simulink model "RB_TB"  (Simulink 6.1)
settings: Solver=ode3  SolverMode=SingleTasking  StartTime=0  StopTime=1000  FixedStep=0.05  RelTol=1e-3
libraries: simulink x2
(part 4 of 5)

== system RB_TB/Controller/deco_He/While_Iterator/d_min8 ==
  note: Model: RB_TB/Controller/deco_He/While_Iterator/d_minX
  Pt_new : Inport  Port=1  LatchInput=off
  In1 : Inport  Port=2  LatchInput=off
  In2 : Inport  Port=3  LatchInput=off
  BC : BusCreator  DialogController=Simulink.DDGSource_Bus
  BS1 : BusSelector  DialogController=Simulink.DDGSource_Bus  OutputSignals=He_b,M0,He_k,Pt
  BS2 : BusSelector  DialogController=Simulink.DDGSource_Bus  OutputSignals=rate_asc,asc_time,while,cnc_He,Palv_next,Palv
  Mux2 : Mux  Inputs=6
  Product2 : Product
  Sum1 : Sum  Inputs=-+|
  Switch : Switch  Threshold=2
  Switch1 : Switch  Threshold=2
  fnc : Fcn  Expr=u(6)-u(5)*u(2)*(u(3)-1/u(1))-(u(6)-u(4)+u(5)*u(2)/u(1))*exp(-u(1)*u(3))
  prod : Gain  Gain=10
  bus1 : Outport
  d_min : Outport  Port=2
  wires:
  BS1/3 -> Mux2/1, BC/3  "<He_k>"
  BS1/1 -> prod/1, BC/1  "<He_b>"
  BS1/2 -> Sum1/1, BC/2  "<M0>"
  Mux2/1 -> fnc/1
  fnc/1 -> BC/4  "Pt_stop"
  BS2/2 -> Mux2/3  "<asc_time>"
  BS2/4 -> Mux2/5  "<cnc_He>"
  In1/1 -> BS1/1
  Sum1/1 -> Product2/2
  prod/1 -> Product2/1
  Product2/1 -> d_min/1
  BC/1 -> bus1/1
  Switch/1 -> Sum1/2, Mux2/4  "Pt"
  BS1/4 -> Switch/3  "<Pt>"
  Pt_new/1 -> Switch/1
  Switch1/1 -> Mux2/6
  BS2/6 -> Switch1/3  "<Palv>"
  BS2/3 -> Switch/2, Switch1/2  "<while>"
  BS2/5 -> Switch1/1  "<Palv_next>"
  In2/1 -> BS2/1
  BS2/1 -> Mux2/2  "<rate_asc>"

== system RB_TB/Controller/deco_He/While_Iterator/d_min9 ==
  note: Model: RB_TB/Controller/deco_He/While_Iterator/d_minX
  Pt_new : Inport  Port=1  LatchInput=off
  In1 : Inport  Port=2  LatchInput=off
  In2 : Inport  Port=3  LatchInput=off
  BC : BusCreator  DialogController=Simulink.DDGSource_Bus
  BS1 : BusSelector  DialogController=Simulink.DDGSource_Bus  OutputSignals=He_b,M0,He_k,Pt
  BS2 : BusSelector  DialogController=Simulink.DDGSource_Bus  OutputSignals=rate_asc,asc_time,while,cnc_He,Palv_next,Palv
  Mux2 : Mux  Inputs=6
  Product2 : Product
  Sum1 : Sum  Inputs=-+|
  Switch : Switch  Threshold=2
  Switch1 : Switch  Threshold=2
  fnc : Fcn  Expr=u(6)-u(5)*u(2)*(u(3)-1/u(1))-(u(6)-u(4)+u(5)*u(2)/u(1))*exp(-u(1)*u(3))
  prod : Gain  Gain=10
  bus1 : Outport
  d_min : Outport  Port=2
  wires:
  BS2/1 -> Mux2/2  "<rate_asc>"
  In2/1 -> BS2/1
  BS2/5 -> Switch1/1  "<Palv_next>"
  BS2/3 -> Switch1/2, Switch/2  "<while>"
  BS2/6 -> Switch1/3  "<Palv>"
  Switch1/1 -> Mux2/6
  Pt_new/1 -> Switch/1
  BS1/4 -> Switch/3  "<Pt>"
  Switch/1 -> Mux2/4, Sum1/2  "Pt"
  BC/1 -> bus1/1
  Product2/1 -> d_min/1
  prod/1 -> Product2/1
  Sum1/1 -> Product2/2
  In1/1 -> BS1/1
  BS2/4 -> Mux2/5  "<cnc_He>"
  BS2/2 -> Mux2/3  "<asc_time>"
  fnc/1 -> BC/4  "Pt_stop"
  Mux2/1 -> fnc/1
  BS1/2 -> BC/2, Sum1/1  "<M0>"
  BS1/1 -> BC/1, prod/1  "<He_b>"
  BS1/3 -> BC/3, Mux2/1  "<He_k>"

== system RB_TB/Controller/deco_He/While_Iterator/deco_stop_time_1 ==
  note: Model: RB_TB/Controller/deco_He/While_Iterator/deco_stop_time_X
  In1 : Inport  Port=1  LatchInput=off
  In2 : Inport  Port=2  LatchInput=off
  >10e-300 : Saturate  UpperLimit=inf  LowerLimit=10e-320
  >10e-320 : Switch  Threshold=10e-320
  BS1 : BusSelector  DialogController=Simulink.DDGSource_Bus  OutputSignals=He_k,Pt_stop,He_b,M0
  BS2 : BusSelector  DialogController=Simulink.DDGSource_Bus  OutputSignals=Pstop_next,Palv_next,stop_time
  Constant : Constant
  Mem : Memory  InheritSampleTime=on
  Mux1 : Mux  Inputs=2
  Mux2 : Mux
  Mux3 : Mux  Inputs=2
  Mux4 : Mux  Inputs=3
  Mux5 : Mux  Inputs=3
  fcn(14)1 : Fcn  Expr=log(u(1))
  fcn(14)2 : Fcn  Expr=u(1)-u(2)
  fcn(14)4 : Fcn  Expr=(u(2)-u(3))/u(1)
  fcn(14)5 : Fcn  Expr=-u(2)/u(1)
  fcn1 : Fcn  Expr=u(2)+u(3)/u(1)
  fcn2 : Fcn  Expr=u(3)+(u(2)-u(3))*exp(-u(1)*u(4))
  Pt_new : Outport
  deco_stop_time : Outport  Port=2
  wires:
  >10e-300/1 -> Mux5/1
  Mux5/1 -> fcn(14)4/1
  fcn(14)2/1 -> >10e-300/1
  Mux3/1 -> fcn(14)2/1
  BS2/1 -> Mux4/3  "<Pstop_next>"
  Constant/1 -> >10e-320/3
  fcn(14)4/1 -> >10e-320/1, >10e-320/2
  fcn(14)1/1 -> Mux1/2
  >10e-320/1 -> fcn(14)1/1
  Mux4/1 -> fcn1/1
  fcn(14)5/1 -> deco_stop_time/1  "deco_stop_time"
  fcn1/1 -> Mux5/2  "M_next"
  BS2/2 -> Mux3/2, Mux5/3, Mux2/3  "<Palv_next>"
  BS1/1 -> Mux1/1, Mux2/1  "<He_k>"
  Mux1/1 -> fcn(14)5/1
  BS1/4 -> Mux4/2  "<M0>"
  BS1/3 -> Mux4/1  "<He_b>"
  In1/1 -> BS1/1
  BS1/2 -> Mux3/1, Mux2/2  "<Pt_stop>"
  Mux2/1 -> fcn2/1
  fcn2/1 -> Mem/1
  BS2/3 -> Mux2/4  "<stop_time>"
  Mem/1 -> Pt_new/1
  In2/1 -> BS2/1

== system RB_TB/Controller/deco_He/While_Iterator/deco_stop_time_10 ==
  note: Model: RB_TB/Controller/deco_He/While_Iterator/deco_stop_time_X
  In1 : Inport  Port=1  LatchInput=off
  In2 : Inport  Port=2  LatchInput=off
  >10e-300 : Saturate  UpperLimit=inf  LowerLimit=10e-320
  >10e-320 : Switch  Threshold=10e-320
  BS1 : BusSelector  DialogController=Simulink.DDGSource_Bus  OutputSignals=He_k,Pt_stop,He_b,M0
  BS2 : BusSelector  DialogController=Simulink.DDGSource_Bus  OutputSignals=Pstop_next,Palv_next,stop_time
  Constant : Constant
  Mem : Memory  InheritSampleTime=on
  Mux1 : Mux  Inputs=2
  Mux2 : Mux
  Mux3 : Mux  Inputs=2
  Mux4 : Mux  Inputs=3
  Mux5 : Mux  Inputs=3
  fcn(14)1 : Fcn  Expr=log(u(1))
  fcn(14)2 : Fcn  Expr=u(1)-u(2)
  fcn(14)4 : Fcn  Expr=(u(2)-u(3))/u(1)
  fcn(14)5 : Fcn  Expr=-u(2)/u(1)
  fcn1 : Fcn  Expr=u(2)+u(3)/u(1)
  fcn2 : Fcn  Expr=u(3)+(u(2)-u(3))*exp(-u(1)*u(4))
  Pt_new : Outport
  deco_stop_time : Outport  Port=2
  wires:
  >10e-300/1 -> Mux5/1
  Mux5/1 -> fcn(14)4/1
  fcn(14)2/1 -> >10e-300/1
  Mux3/1 -> fcn(14)2/1
  BS2/1 -> Mux4/3  "<Pstop_next>"
  Constant/1 -> >10e-320/3
  fcn(14)4/1 -> >10e-320/1, >10e-320/2
  fcn(14)1/1 -> Mux1/2
  >10e-320/1 -> fcn(14)1/1
  Mux4/1 -> fcn1/1
  fcn(14)5/1 -> deco_stop_time/1  "deco_stop_time"
  fcn1/1 -> Mux5/2  "M_next"
  BS2/2 -> Mux3/2, Mux5/3, Mux2/3  "<Palv_next>"
  BS1/1 -> Mux1/1, Mux2/1  "<He_k>"
  Mux1/1 -> fcn(14)5/1
  BS1/4 -> Mux4/2  "<M0>"
  BS1/3 -> Mux4/1  "<He_b>"
  In1/1 -> BS1/1
  BS1/2 -> Mux3/1, Mux2/2  "<Pt_stop>"
  Mux2/1 -> fcn2/1
  fcn2/1 -> Mem/1
  BS2/3 -> Mux2/4  "<stop_time>"
  Mem/1 -> Pt_new/1
  In2/1 -> BS2/1

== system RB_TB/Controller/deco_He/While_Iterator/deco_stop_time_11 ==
  note: Model: RB_TB/Controller/deco_He/While_Iterator/deco_stop_time_X
  In1 : Inport  Port=1  LatchInput=off
  In2 : Inport  Port=2  LatchInput=off
  >10e-300 : Saturate  UpperLimit=inf  LowerLimit=10e-320
  >10e-320 : Switch  Threshold=10e-320
  BS1 : BusSelector  DialogController=Simulink.DDGSource_Bus  OutputSignals=He_k,Pt_stop,He_b,M0
  BS2 : BusSelector  DialogController=Simulink.DDGSource_Bus  OutputSignals=Pstop_next,Palv_next,stop_time
  Constant : Constant
  Mem : Memory  InheritSampleTime=on
  Mux1 : Mux  Inputs=2
  Mux2 : Mux
  Mux3 : Mux  Inputs=2
  Mux4 : Mux  Inputs=3
  Mux5 : Mux  Inputs=3
  fcn(14)1 : Fcn  Expr=log(u(1))
  fcn(14)2 : Fcn  Expr=u(1)-u(2)
  fcn(14)4 : Fcn  Expr=(u(2)-u(3))/u(1)
  fcn(14)5 : Fcn  Expr=-u(2)/u(1)
  fcn1 : Fcn  Expr=u(2)+u(3)/u(1)
  fcn2 : Fcn  Expr=u(3)+(u(2)-u(3))*exp(-u(1)*u(4))
  Pt_new : Outport
  deco_stop_time : Outport  Port=2
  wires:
  In2/1 -> BS2/1
  Mem/1 -> Pt_new/1
  BS2/3 -> Mux2/4  "<stop_time>"
  fcn2/1 -> Mem/1
  Mux2/1 -> fcn2/1
  BS1/2 -> Mux2/2, Mux3/1  "<Pt_stop>"
  In1/1 -> BS1/1
  BS1/3 -> Mux4/1  "<He_b>"
  BS1/4 -> Mux4/2  "<M0>"
  Mux1/1 -> fcn(14)5/1
  BS1/1 -> Mux2/1, Mux1/1  "<He_k>"
  BS2/2 -> Mux2/3, Mux5/3, Mux3/2  "<Palv_next>"
  fcn1/1 -> Mux5/2  "M_next"
  fcn(14)5/1 -> deco_stop_time/1  "deco_stop_time"
  Mux4/1 -> fcn1/1
  >10e-320/1 -> fcn(14)1/1
  fcn(14)1/1 -> Mux1/2
  fcn(14)4/1 -> >10e-320/2, >10e-320/1
  Constant/1 -> >10e-320/3
  BS2/1 -> Mux4/3  "<Pstop_next>"
  Mux3/1 -> fcn(14)2/1
  fcn(14)2/1 -> >10e-300/1
  Mux5/1 -> fcn(14)4/1
  >10e-300/1 -> Mux5/1

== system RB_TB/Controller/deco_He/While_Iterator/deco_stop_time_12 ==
  note: Model: RB_TB/Controller/deco_He/While_Iterator/deco_stop_time_X
  In1 : Inport  Port=1  LatchInput=off
  In2 : Inport  Port=2  LatchInput=off
  >10e-300 : Saturate  UpperLimit=inf  LowerLimit=10e-320
  >10e-320 : Switch  Threshold=10e-320
  BS1 : BusSelector  DialogController=Simulink.DDGSource_Bus  OutputSignals=He_k,Pt_stop,He_b,M0
  BS2 : BusSelector  DialogController=Simulink.DDGSource_Bus  OutputSignals=Pstop_next,Palv_next,stop_time
  Constant : Constant
  Mem : Memory  InheritSampleTime=on
  Mux1 : Mux  Inputs=2
  Mux2 : Mux
  Mux3 : Mux  Inputs=2
  Mux4 : Mux  Inputs=3
  Mux5 : Mux  Inputs=3
  fcn(14)1 : Fcn  Expr=log(u(1))
  fcn(14)2 : Fcn  Expr=u(1)-u(2)
  fcn(14)4 : Fcn  Expr=(u(2)-u(3))/u(1)
  fcn(14)5 : Fcn  Expr=-u(2)/u(1)
  fcn1 : Fcn  Expr=u(2)+u(3)/u(1)
  fcn2 : Fcn  Expr=u(3)+(u(2)-u(3))*exp(-u(1)*u(4))
  Pt_new : Outport
  deco_stop_time : Outport  Port=2
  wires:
  >10e-300/1 -> Mux5/1
  Mux5/1 -> fcn(14)4/1
  fcn(14)2/1 -> >10e-300/1
  Mux3/1 -> fcn(14)2/1
  BS2/1 -> Mux4/3  "<Pstop_next>"
  Constant/1 -> >10e-320/3
  fcn(14)4/1 -> >10e-320/1, >10e-320/2
  fcn(14)1/1 -> Mux1/2
  >10e-320/1 -> fcn(14)1/1
  Mux4/1 -> fcn1/1
  fcn(14)5/1 -> deco_stop_time/1  "deco_stop_time"
  fcn1/1 -> Mux5/2  "M_next"
  BS2/2 -> Mux3/2, Mux5/3, Mux2/3  "<Palv_next>"
  BS1/1 -> Mux1/1, Mux2/1  "<He_k>"
  Mux1/1 -> fcn(14)5/1
  BS1/4 -> Mux4/2  "<M0>"
  BS1/3 -> Mux4/1  "<He_b>"
  In1/1 -> BS1/1
  BS1/2 -> Mux3/1, Mux2/2  "<Pt_stop>"
  Mux2/1 -> fcn2/1
  fcn2/1 -> Mem/1
  BS2/3 -> Mux2/4  "<stop_time>"
  Mem/1 -> Pt_new/1
  In2/1 -> BS2/1

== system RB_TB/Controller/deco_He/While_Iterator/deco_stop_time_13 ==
  note: Model: RB_TB/Controller/deco_He/While_Iterator/deco_stop_time_X
  In1 : Inport  Port=1  LatchInput=off
  In2 : Inport  Port=2  LatchInput=off
  >10e-300 : Saturate  UpperLimit=inf  LowerLimit=10e-320
  >10e-320 : Switch  Threshold=10e-320
  BS1 : BusSelector  DialogController=Simulink.DDGSource_Bus  OutputSignals=He_k,Pt_stop,He_b,M0
  BS2 : BusSelector  DialogController=Simulink.DDGSource_Bus  OutputSignals=Pstop_next,Palv_next,stop_time
  Constant : Constant
  Mem : Memory  InheritSampleTime=on
  Mux1 : Mux  Inputs=2
  Mux2 : Mux
  Mux3 : Mux  Inputs=2
  Mux4 : Mux  Inputs=3
  Mux5 : Mux  Inputs=3
  fcn(14)1 : Fcn  Expr=log(u(1))
  fcn(14)2 : Fcn  Expr=u(1)-u(2)
  fcn(14)4 : Fcn  Expr=(u(2)-u(3))/u(1)
  fcn(14)5 : Fcn  Expr=-u(2)/u(1)
  fcn1 : Fcn  Expr=u(2)+u(3)/u(1)
  fcn2 : Fcn  Expr=u(3)+(u(2)-u(3))*exp(-u(1)*u(4))
  Pt_new : Outport
  deco_stop_time : Outport  Port=2
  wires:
  In2/1 -> BS2/1
  Mem/1 -> Pt_new/1
  BS2/3 -> Mux2/4  "<stop_time>"
  fcn2/1 -> Mem/1
  Mux2/1 -> fcn2/1
  BS1/2 -> Mux2/2, Mux3/1  "<Pt_stop>"
  In1/1 -> BS1/1
  BS1/3 -> Mux4/1  "<He_b>"
  BS1/4 -> Mux4/2  "<M0>"
  Mux1/1 -> fcn(14)5/1
  BS1/1 -> Mux2/1, Mux1/1  "<He_k>"
  BS2/2 -> Mux2/3, Mux5/3, Mux3/2  "<Palv_next>"
  fcn1/1 -> Mux5/2  "M_next"
  fcn(14)5/1 -> deco_stop_time/1  "deco_stop_time"
  Mux4/1 -> fcn1/1
  >10e-320/1 -> fcn(14)1/1
  fcn(14)1/1 -> Mux1/2
  fcn(14)4/1 -> >10e-320/2, >10e-320/1
  Constant/1 -> >10e-320/3
  BS2/1 -> Mux4/3  "<Pstop_next>"
  Mux3/1 -> fcn(14)2/1
  fcn(14)2/1 -> >10e-300/1
  Mux5/1 -> fcn(14)4/1
  >10e-300/1 -> Mux5/1

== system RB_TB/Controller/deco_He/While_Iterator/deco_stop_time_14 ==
  note: Model: RB_TB/Controller/deco_He/While_Iterator/deco_stop_time_X
  In1 : Inport  Port=1  LatchInput=off
  In2 : Inport  Port=2  LatchInput=off
  >10e-300 : Saturate  UpperLimit=inf  LowerLimit=10e-320
  >10e-320 : Switch  Threshold=10e-320
  BS1 : BusSelector  DialogController=Simulink.DDGSource_Bus  OutputSignals=He_k,Pt_stop,He_b,M0
  BS2 : BusSelector  DialogController=Simulink.DDGSource_Bus  OutputSignals=Pstop_next,Palv_next,stop_time
  Constant : Constant
  Mem : Memory  InheritSampleTime=on
  Mux1 : Mux  Inputs=2
  Mux2 : Mux
  Mux3 : Mux  Inputs=2
  Mux4 : Mux  Inputs=3
  Mux5 : Mux  Inputs=3
  fcn(14)1 : Fcn  Expr=log(u(1))
  fcn(14)2 : Fcn  Expr=u(1)-u(2)
  fcn(14)4 : Fcn  Expr=(u(2)-u(3))/u(1)
  fcn(14)5 : Fcn  Expr=-u(2)/u(1)
  fcn1 : Fcn  Expr=u(2)+u(3)/u(1)
  fcn2 : Fcn  Expr=u(3)+(u(2)-u(3))*exp(-u(1)*u(4))
  Pt_new : Outport
  deco_stop_time : Outport  Port=2
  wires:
  >10e-300/1 -> Mux5/1
  Mux5/1 -> fcn(14)4/1
  fcn(14)2/1 -> >10e-300/1
  Mux3/1 -> fcn(14)2/1
  BS2/1 -> Mux4/3  "<Pstop_next>"
  Constant/1 -> >10e-320/3
  fcn(14)4/1 -> >10e-320/1, >10e-320/2
  fcn(14)1/1 -> Mux1/2
  >10e-320/1 -> fcn(14)1/1
  Mux4/1 -> fcn1/1
  fcn(14)5/1 -> deco_stop_time/1  "deco_stop_time"
  fcn1/1 -> Mux5/2  "M_next"
  BS2/2 -> Mux3/2, Mux5/3, Mux2/3  "<Palv_next>"
  BS1/1 -> Mux1/1, Mux2/1  "<He_k>"
  Mux1/1 -> fcn(14)5/1
  BS1/4 -> Mux4/2  "<M0>"
  BS1/3 -> Mux4/1  "<He_b>"
  In1/1 -> BS1/1
  BS1/2 -> Mux3/1, Mux2/2  "<Pt_stop>"
  Mux2/1 -> fcn2/1
  fcn2/1 -> Mem/1
  BS2/3 -> Mux2/4  "<stop_time>"
  Mem/1 -> Pt_new/1
  In2/1 -> BS2/1

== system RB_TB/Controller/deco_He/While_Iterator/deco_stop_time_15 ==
  note: Model: RB_TB/Controller/deco_He/While_Iterator/deco_stop_time_X
  In1 : Inport  Port=1  LatchInput=off
  In2 : Inport  Port=2  LatchInput=off
  >10e-300 : Saturate  UpperLimit=inf  LowerLimit=10e-320
  >10e-320 : Switch  Threshold=10e-320
  BS1 : BusSelector  DialogController=Simulink.DDGSource_Bus  OutputSignals=He_k,Pt_stop,He_b,M0
  BS2 : BusSelector  DialogController=Simulink.DDGSource_Bus  OutputSignals=Pstop_next,Palv_next,stop_time
  Constant : Constant
  Mem : Memory  InheritSampleTime=on
  Mux1 : Mux  Inputs=2
  Mux2 : Mux
  Mux3 : Mux  Inputs=2
  Mux4 : Mux  Inputs=3
  Mux5 : Mux  Inputs=3
  fcn(14)1 : Fcn  Expr=log(u(1))
  fcn(14)2 : Fcn  Expr=u(1)-u(2)
  fcn(14)4 : Fcn  Expr=(u(2)-u(3))/u(1)
  fcn(14)5 : Fcn  Expr=-u(2)/u(1)
  fcn1 : Fcn  Expr=u(2)+u(3)/u(1)
  fcn2 : Fcn  Expr=u(3)+(u(2)-u(3))*exp(-u(1)*u(4))
  Pt_new : Outport
  deco_stop_time : Outport  Port=2
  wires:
  In2/1 -> BS2/1
  Mem/1 -> Pt_new/1
  BS2/3 -> Mux2/4  "<stop_time>"
  fcn2/1 -> Mem/1
  Mux2/1 -> fcn2/1
  BS1/2 -> Mux2/2, Mux3/1  "<Pt_stop>"
  In1/1 -> BS1/1
  BS1/3 -> Mux4/1  "<He_b>"
  BS1/4 -> Mux4/2  "<M0>"
  Mux1/1 -> fcn(14)5/1
  BS1/1 -> Mux2/1, Mux1/1  "<He_k>"
  BS2/2 -> Mux2/3, Mux5/3, Mux3/2  "<Palv_next>"
  fcn1/1 -> Mux5/2  "M_next"
  fcn(14)5/1 -> deco_stop_time/1  "deco_stop_time"
  Mux4/1 -> fcn1/1
  >10e-320/1 -> fcn(14)1/1
  fcn(14)1/1 -> Mux1/2
  fcn(14)4/1 -> >10e-320/2, >10e-320/1
  Constant/1 -> >10e-320/3
  BS2/1 -> Mux4/3  "<Pstop_next>"
  Mux3/1 -> fcn(14)2/1
  fcn(14)2/1 -> >10e-300/1
  Mux5/1 -> fcn(14)4/1
  >10e-300/1 -> Mux5/1

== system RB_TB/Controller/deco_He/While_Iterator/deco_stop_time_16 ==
  note: Model: RB_TB/Controller/deco_He/While_Iterator/deco_stop_time_X
  In1 : Inport  Port=1  LatchInput=off
  In2 : Inport  Port=2  LatchInput=off
  >10e-300 : Saturate  UpperLimit=inf  LowerLimit=10e-320
  >10e-320 : Switch  Threshold=10e-320
  BS1 : BusSelector  DialogController=Simulink.DDGSource_Bus  OutputSignals=He_k,Pt_stop,He_b,M0
  BS2 : BusSelector  DialogController=Simulink.DDGSource_Bus  OutputSignals=Pstop_next,Palv_next,stop_time
  Constant : Constant
  Mem : Memory  InheritSampleTime=on
  Mux1 : Mux  Inputs=2
  Mux2 : Mux
  Mux3 : Mux  Inputs=2
  Mux4 : Mux  Inputs=3
  Mux5 : Mux  Inputs=3
  fcn(14)1 : Fcn  Expr=log(u(1))
  fcn(14)2 : Fcn  Expr=u(1)-u(2)
  fcn(14)4 : Fcn  Expr=(u(2)-u(3))/u(1)
  fcn(14)5 : Fcn  Expr=-u(2)/u(1)
  fcn1 : Fcn  Expr=u(2)+u(3)/u(1)
  fcn2 : Fcn  Expr=u(3)+(u(2)-u(3))*exp(-u(1)*u(4))
  Pt_new : Outport
  deco_stop_time : Outport  Port=2
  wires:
  >10e-300/1 -> Mux5/1
  Mux5/1 -> fcn(14)4/1
  fcn(14)2/1 -> >10e-300/1
  Mux3/1 -> fcn(14)2/1
  BS2/1 -> Mux4/3  "<Pstop_next>"
  Constant/1 -> >10e-320/3
  fcn(14)4/1 -> >10e-320/1, >10e-320/2
  fcn(14)1/1 -> Mux1/2
  >10e-320/1 -> fcn(14)1/1
  Mux4/1 -> fcn1/1
  fcn(14)5/1 -> deco_stop_time/1  "deco_stop_time"
  fcn1/1 -> Mux5/2  "M_next"
  BS2/2 -> Mux3/2, Mux5/3, Mux2/3  "<Palv_next>"
  BS1/1 -> Mux1/1, Mux2/1  "<He_k>"
  Mux1/1 -> fcn(14)5/1
  BS1/4 -> Mux4/2  "<M0>"
  BS1/3 -> Mux4/1  "<He_b>"
  In1/1 -> BS1/1
  BS1/2 -> Mux3/1, Mux2/2  "<Pt_stop>"
  Mux2/1 -> fcn2/1
  fcn2/1 -> Mem/1
  BS2/3 -> Mux2/4  "<stop_time>"
  Mem/1 -> Pt_new/1
  In2/1 -> BS2/1

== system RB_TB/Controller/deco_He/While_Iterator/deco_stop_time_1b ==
  note: Model: RB_TB/Controller/deco_He/While_Iterator/deco_stop_time_X
  In1 : Inport  Port=1  LatchInput=off
  In2 : Inport  Port=2  LatchInput=off
  >10e-300 : Saturate  UpperLimit=inf  LowerLimit=10e-320
  >10e-320 : Switch  Threshold=10e-320
  BS1 : BusSelector  DialogController=Simulink.DDGSource_Bus  OutputSignals=He_k,Pt_stop,He_b,M0
  BS2 : BusSelector  DialogController=Simulink.DDGSource_Bus  OutputSignals=Pstop_next,Palv_next,stop_time
  Constant : Constant
  Mem : Memory  InheritSampleTime=on
  Mux1 : Mux  Inputs=2
  Mux2 : Mux
  Mux3 : Mux  Inputs=2
  Mux4 : Mux  Inputs=3
  Mux5 : Mux  Inputs=3
  fcn(14)1 : Fcn  Expr=log(u(1))
  fcn(14)2 : Fcn  Expr=u(1)-u(2)
  fcn(14)4 : Fcn  Expr=(u(2)-u(3))/u(1)
  fcn(14)5 : Fcn  Expr=-u(2)/u(1)
  fcn1 : Fcn  Expr=u(2)+u(3)/u(1)
  fcn2 : Fcn  Expr=u(3)+(u(2)-u(3))*exp(-u(1)*u(4))
  Pt_new : Outport
  deco_stop_time : Outport  Port=2
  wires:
  >10e-300/1 -> Mux5/1
  Mux5/1 -> fcn(14)4/1
  fcn(14)2/1 -> >10e-300/1
  Mux3/1 -> fcn(14)2/1
  BS2/1 -> Mux4/3  "<Pstop_next>"
  Constant/1 -> >10e-320/3
  fcn(14)4/1 -> >10e-320/1, >10e-320/2
  fcn(14)1/1 -> Mux1/2
  >10e-320/1 -> fcn(14)1/1
  Mux4/1 -> fcn1/1
  fcn(14)5/1 -> deco_stop_time/1  "deco_stop_time"
  fcn1/1 -> Mux5/2  "M_next"
  BS2/2 -> Mux3/2, Mux5/3, Mux2/3  "<Palv_next>"
  BS1/1 -> Mux1/1, Mux2/1  "<He_k>"
  Mux1/1 -> fcn(14)5/1
  BS1/4 -> Mux4/2  "<M0>"
  BS1/3 -> Mux4/1  "<He_b>"
  In1/1 -> BS1/1
  BS1/2 -> Mux3/1, Mux2/2  "<Pt_stop>"
  Mux2/1 -> fcn2/1
  fcn2/1 -> Mem/1
  BS2/3 -> Mux2/4  "<stop_time>"
  Mem/1 -> Pt_new/1
  In2/1 -> BS2/1

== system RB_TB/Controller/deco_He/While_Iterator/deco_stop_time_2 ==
  note: Model: RB_TB/Controller/deco_He/While_Iterator/deco_stop_time_X
  In1 : Inport  Port=1  LatchInput=off
  In2 : Inport  Port=2  LatchInput=off
  >10e-300 : Saturate  UpperLimit=inf  LowerLimit=10e-320
  >10e-320 : Switch  Threshold=10e-320
  BS1 : BusSelector  DialogController=Simulink.DDGSource_Bus  OutputSignals=He_k,Pt_stop,He_b,M0
  BS2 : BusSelector  DialogController=Simulink.DDGSource_Bus  OutputSignals=Pstop_next,Palv_next,stop_time
  Constant : Constant
  Mem : Memory  InheritSampleTime=on
  Mux1 : Mux  Inputs=2
  Mux2 : Mux
  Mux3 : Mux  Inputs=2
  Mux4 : Mux  Inputs=3
  Mux5 : Mux  Inputs=3
  fcn(14)1 : Fcn  Expr=log(u(1))
  fcn(14)2 : Fcn  Expr=u(1)-u(2)
  fcn(14)4 : Fcn  Expr=(u(2)-u(3))/u(1)
  fcn(14)5 : Fcn  Expr=-u(2)/u(1)
  fcn1 : Fcn  Expr=u(2)+u(3)/u(1)
  fcn2 : Fcn  Expr=u(3)+(u(2)-u(3))*exp(-u(1)*u(4))
  Pt_new : Outport
  deco_stop_time : Outport  Port=2
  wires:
  In2/1 -> BS2/1
  Mem/1 -> Pt_new/1
  BS2/3 -> Mux2/4  "<stop_time>"
  fcn2/1 -> Mem/1
  Mux2/1 -> fcn2/1
  BS1/2 -> Mux2/2, Mux3/1  "<Pt_stop>"
  In1/1 -> BS1/1
  BS1/3 -> Mux4/1  "<He_b>"
  BS1/4 -> Mux4/2  "<M0>"
  Mux1/1 -> fcn(14)5/1
  BS1/1 -> Mux2/1, Mux1/1  "<He_k>"
  BS2/2 -> Mux2/3, Mux5/3, Mux3/2  "<Palv_next>"
  fcn1/1 -> Mux5/2  "M_next"
  fcn(14)5/1 -> deco_stop_time/1  "deco_stop_time"
  Mux4/1 -> fcn1/1
  >10e-320/1 -> fcn(14)1/1
  fcn(14)1/1 -> Mux1/2
  fcn(14)4/1 -> >10e-320/2, >10e-320/1
  Constant/1 -> >10e-320/3
  BS2/1 -> Mux4/3  "<Pstop_next>"
  Mux3/1 -> fcn(14)2/1
  fcn(14)2/1 -> >10e-300/1
  Mux5/1 -> fcn(14)4/1
  >10e-300/1 -> Mux5/1

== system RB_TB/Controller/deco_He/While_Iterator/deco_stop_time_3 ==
  note: Model: RB_TB/Controller/deco_He/While_Iterator/deco_stop_time_X
  In1 : Inport  Port=1  LatchInput=off
  In2 : Inport  Port=2  LatchInput=off
  >10e-300 : Saturate  UpperLimit=inf  LowerLimit=10e-320
  >10e-320 : Switch  Threshold=10e-320
  BS1 : BusSelector  DialogController=Simulink.DDGSource_Bus  OutputSignals=He_k,Pt_stop,He_b,M0
  BS2 : BusSelector  DialogController=Simulink.DDGSource_Bus  OutputSignals=Pstop_next,Palv_next,stop_time
  Constant : Constant
  Mem : Memory  InheritSampleTime=on
  Mux1 : Mux  Inputs=2
  Mux2 : Mux
  Mux3 : Mux  Inputs=2
  Mux4 : Mux  Inputs=3
  Mux5 : Mux  Inputs=3
  fcn(14)1 : Fcn  Expr=log(u(1))
  fcn(14)2 : Fcn  Expr=u(1)-u(2)
  fcn(14)4 : Fcn  Expr=(u(2)-u(3))/u(1)
  fcn(14)5 : Fcn  Expr=-u(2)/u(1)
  fcn1 : Fcn  Expr=u(2)+u(3)/u(1)
  fcn2 : Fcn  Expr=u(3)+(u(2)-u(3))*exp(-u(1)*u(4))
  Pt_new : Outport
  deco_stop_time : Outport  Port=2
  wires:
  In2/1 -> BS2/1
  Mem/1 -> Pt_new/1
  BS2/3 -> Mux2/4  "<stop_time>"
  fcn2/1 -> Mem/1
  Mux2/1 -> fcn2/1
  BS1/2 -> Mux2/2, Mux3/1  "<Pt_stop>"
  In1/1 -> BS1/1
  BS1/3 -> Mux4/1  "<He_b>"
  BS1/4 -> Mux4/2  "<M0>"
  Mux1/1 -> fcn(14)5/1
  BS1/1 -> Mux2/1, Mux1/1  "<He_k>"
  BS2/2 -> Mux2/3, Mux5/3, Mux3/2  "<Palv_next>"
  fcn1/1 -> Mux5/2  "M_next"
  fcn(14)5/1 -> deco_stop_time/1  "deco_stop_time"
  Mux4/1 -> fcn1/1
  >10e-320/1 -> fcn(14)1/1
  fcn(14)1/1 -> Mux1/2
  fcn(14)4/1 -> >10e-320/2, >10e-320/1
  Constant/1 -> >10e-320/3
  BS2/1 -> Mux4/3  "<Pstop_next>"
  Mux3/1 -> fcn(14)2/1
  fcn(14)2/1 -> >10e-300/1
  Mux5/1 -> fcn(14)4/1
  >10e-300/1 -> Mux5/1

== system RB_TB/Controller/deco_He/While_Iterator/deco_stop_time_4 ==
  note: Model: RB_TB/Controller/deco_He/While_Iterator/deco_stop_time_X
  In1 : Inport  Port=1  LatchInput=off
  In2 : Inport  Port=2  LatchInput=off
  >10e-300 : Saturate  UpperLimit=inf  LowerLimit=10e-320
  >10e-320 : Switch  Threshold=10e-320
  BS1 : BusSelector  DialogController=Simulink.DDGSource_Bus  OutputSignals=He_k,Pt_stop,He_b,M0
  BS2 : BusSelector  DialogController=Simulink.DDGSource_Bus  OutputSignals=Pstop_next,Palv_next,stop_time
  Constant : Constant
  Mem : Memory  InheritSampleTime=on
  Mux1 : Mux  Inputs=2
  Mux2 : Mux
  Mux3 : Mux  Inputs=2
  Mux4 : Mux  Inputs=3
  Mux5 : Mux  Inputs=3
  fcn(14)1 : Fcn  Expr=log(u(1))
  fcn(14)2 : Fcn  Expr=u(1)-u(2)
  fcn(14)4 : Fcn  Expr=(u(2)-u(3))/u(1)
  fcn(14)5 : Fcn  Expr=-u(2)/u(1)
  fcn1 : Fcn  Expr=u(2)+u(3)/u(1)
  fcn2 : Fcn  Expr=u(3)+(u(2)-u(3))*exp(-u(1)*u(4))
  Pt_new : Outport
  deco_stop_time : Outport  Port=2
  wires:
  >10e-300/1 -> Mux5/1
  Mux5/1 -> fcn(14)4/1
  fcn(14)2/1 -> >10e-300/1
  Mux3/1 -> fcn(14)2/1
  BS2/1 -> Mux4/3  "<Pstop_next>"
  Constant/1 -> >10e-320/3
  fcn(14)4/1 -> >10e-320/1, >10e-320/2
  fcn(14)1/1 -> Mux1/2
  >10e-320/1 -> fcn(14)1/1
  Mux4/1 -> fcn1/1
  fcn(14)5/1 -> deco_stop_time/1  "deco_stop_time"
  fcn1/1 -> Mux5/2  "M_next"
  BS2/2 -> Mux3/2, Mux5/3, Mux2/3  "<Palv_next>"
  BS1/1 -> Mux1/1, Mux2/1  "<He_k>"
  Mux1/1 -> fcn(14)5/1
  BS1/4 -> Mux4/2  "<M0>"
  BS1/3 -> Mux4/1  "<He_b>"
  In1/1 -> BS1/1
  BS1/2 -> Mux3/1, Mux2/2  "<Pt_stop>"
  Mux2/1 -> fcn2/1
  fcn2/1 -> Mem/1
  BS2/3 -> Mux2/4  "<stop_time>"
  Mem/1 -> Pt_new/1
  In2/1 -> BS2/1

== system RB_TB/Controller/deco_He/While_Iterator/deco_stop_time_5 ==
  note: Model: RB_TB/Controller/deco_He/While_Iterator/deco_stop_time_X
  In1 : Inport  Port=1  LatchInput=off
  In2 : Inport  Port=2  LatchInput=off
  >10e-300 : Saturate  UpperLimit=inf  LowerLimit=10e-320
  >10e-320 : Switch  Threshold=10e-320
  BS1 : BusSelector  DialogController=Simulink.DDGSource_Bus  OutputSignals=He_k,Pt_stop,He_b,M0
  BS2 : BusSelector  DialogController=Simulink.DDGSource_Bus  OutputSignals=Pstop_next,Palv_next,stop_time
  Constant : Constant
  Mem : Memory  InheritSampleTime=on
  Mux1 : Mux  Inputs=2
  Mux2 : Mux
  Mux3 : Mux  Inputs=2
  Mux4 : Mux  Inputs=3
  Mux5 : Mux  Inputs=3
  fcn(14)1 : Fcn  Expr=log(u(1))
  fcn(14)2 : Fcn  Expr=u(1)-u(2)
  fcn(14)4 : Fcn  Expr=(u(2)-u(3))/u(1)
  fcn(14)5 : Fcn  Expr=-u(2)/u(1)
  fcn1 : Fcn  Expr=u(2)+u(3)/u(1)
  fcn2 : Fcn  Expr=u(3)+(u(2)-u(3))*exp(-u(1)*u(4))
  Pt_new : Outport
  deco_stop_time : Outport  Port=2
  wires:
  In2/1 -> BS2/1
  Mem/1 -> Pt_new/1
  BS2/3 -> Mux2/4  "<stop_time>"
  fcn2/1 -> Mem/1
  Mux2/1 -> fcn2/1
  BS1/2 -> Mux2/2, Mux3/1  "<Pt_stop>"
  In1/1 -> BS1/1
  BS1/3 -> Mux4/1  "<He_b>"
  BS1/4 -> Mux4/2  "<M0>"
  Mux1/1 -> fcn(14)5/1
  BS1/1 -> Mux2/1, Mux1/1  "<He_k>"
  BS2/2 -> Mux2/3, Mux5/3, Mux3/2  "<Palv_next>"
  fcn1/1 -> Mux5/2  "M_next"
  fcn(14)5/1 -> deco_stop_time/1  "deco_stop_time"
  Mux4/1 -> fcn1/1
  >10e-320/1 -> fcn(14)1/1
  fcn(14)1/1 -> Mux1/2
  fcn(14)4/1 -> >10e-320/2, >10e-320/1
  Constant/1 -> >10e-320/3
  BS2/1 -> Mux4/3  "<Pstop_next>"
  Mux3/1 -> fcn(14)2/1
  fcn(14)2/1 -> >10e-300/1
  Mux5/1 -> fcn(14)4/1
  >10e-300/1 -> Mux5/1

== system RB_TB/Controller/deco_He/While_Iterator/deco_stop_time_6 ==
  note: Model: RB_TB/Controller/deco_He/While_Iterator/deco_stop_time_X
  In1 : Inport  Port=1  LatchInput=off
  In2 : Inport  Port=2  LatchInput=off
  >10e-300 : Saturate  UpperLimit=inf  LowerLimit=10e-320
  >10e-320 : Switch  Threshold=10e-320
  BS1 : BusSelector  DialogController=Simulink.DDGSource_Bus  OutputSignals=He_k,Pt_stop,He_b,M0
  BS2 : BusSelector  DialogController=Simulink.DDGSource_Bus  OutputSignals=Pstop_next,Palv_next,stop_time
  Constant : Constant
  Mem : Memory  InheritSampleTime=on
  Mux1 : Mux  Inputs=2
  Mux2 : Mux
  Mux3 : Mux  Inputs=2
  Mux4 : Mux  Inputs=3
  Mux5 : Mux  Inputs=3
  fcn(14)1 : Fcn  Expr=log(u(1))
  fcn(14)2 : Fcn  Expr=u(1)-u(2)
  fcn(14)4 : Fcn  Expr=(u(2)-u(3))/u(1)
  fcn(14)5 : Fcn  Expr=-u(2)/u(1)
  fcn1 : Fcn  Expr=u(2)+u(3)/u(1)
  fcn2 : Fcn  Expr=u(3)+(u(2)-u(3))*exp(-u(1)*u(4))
  Pt_new : Outport
  deco_stop_time : Outport  Port=2
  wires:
  >10e-300/1 -> Mux5/1
  Mux5/1 -> fcn(14)4/1
  fcn(14)2/1 -> >10e-300/1
  Mux3/1 -> fcn(14)2/1
  BS2/1 -> Mux4/3  "<Pstop_next>"
  Constant/1 -> >10e-320/3
  fcn(14)4/1 -> >10e-320/1, >10e-320/2
  fcn(14)1/1 -> Mux1/2
  >10e-320/1 -> fcn(14)1/1
  Mux4/1 -> fcn1/1
  fcn(14)5/1 -> deco_stop_time/1  "deco_stop_time"
  fcn1/1 -> Mux5/2  "M_next"
  BS2/2 -> Mux3/2, Mux5/3, Mux2/3  "<Palv_next>"
  BS1/1 -> Mux1/1, Mux2/1  "<He_k>"
  Mux1/1 -> fcn(14)5/1
  BS1/4 -> Mux4/2  "<M0>"
  BS1/3 -> Mux4/1  "<He_b>"
  In1/1 -> BS1/1
  BS1/2 -> Mux3/1, Mux2/2  "<Pt_stop>"
  Mux2/1 -> fcn2/1
  fcn2/1 -> Mem/1
  BS2/3 -> Mux2/4  "<stop_time>"
  Mem/1 -> Pt_new/1
  In2/1 -> BS2/1

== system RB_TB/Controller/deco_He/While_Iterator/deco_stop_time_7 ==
  note: Model: RB_TB/Controller/deco_He/While_Iterator/deco_stop_time_X
  In1 : Inport  Port=1  LatchInput=off
  In2 : Inport  Port=2  LatchInput=off
  >10e-300 : Saturate  UpperLimit=inf  LowerLimit=10e-320
  >10e-320 : Switch  Threshold=10e-320
  BS1 : BusSelector  DialogController=Simulink.DDGSource_Bus  OutputSignals=He_k,Pt_stop,He_b,M0
  BS2 : BusSelector  DialogController=Simulink.DDGSource_Bus  OutputSignals=Pstop_next,Palv_next,stop_time
  Constant : Constant
  Mem : Memory  InheritSampleTime=on
  Mux1 : Mux  Inputs=2
  Mux2 : Mux
  Mux3 : Mux  Inputs=2
  Mux4 : Mux  Inputs=3
  Mux5 : Mux  Inputs=3
  fcn(14)1 : Fcn  Expr=log(u(1))
  fcn(14)2 : Fcn  Expr=u(1)-u(2)
  fcn(14)4 : Fcn  Expr=(u(2)-u(3))/u(1)
  fcn(14)5 : Fcn  Expr=-u(2)/u(1)
  fcn1 : Fcn  Expr=u(2)+u(3)/u(1)
  fcn2 : Fcn  Expr=u(3)+(u(2)-u(3))*exp(-u(1)*u(4))
  Pt_new : Outport
  deco_stop_time : Outport  Port=2
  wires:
  In2/1 -> BS2/1
  Mem/1 -> Pt_new/1
  BS2/3 -> Mux2/4  "<stop_time>"
  fcn2/1 -> Mem/1
  Mux2/1 -> fcn2/1
  BS1/2 -> Mux2/2, Mux3/1  "<Pt_stop>"
  In1/1 -> BS1/1
  BS1/3 -> Mux4/1  "<He_b>"
  BS1/4 -> Mux4/2  "<M0>"
  Mux1/1 -> fcn(14)5/1
  BS1/1 -> Mux2/1, Mux1/1  "<He_k>"
  BS2/2 -> Mux2/3, Mux5/3, Mux3/2  "<Palv_next>"
  fcn1/1 -> Mux5/2  "M_next"
  fcn(14)5/1 -> deco_stop_time/1  "deco_stop_time"
  Mux4/1 -> fcn1/1
  >10e-320/1 -> fcn(14)1/1
  fcn(14)1/1 -> Mux1/2
  fcn(14)4/1 -> >10e-320/2, >10e-320/1
  Constant/1 -> >10e-320/3
  BS2/1 -> Mux4/3  "<Pstop_next>"
  Mux3/1 -> fcn(14)2/1
  fcn(14)2/1 -> >10e-300/1
  Mux5/1 -> fcn(14)4/1
  >10e-300/1 -> Mux5/1

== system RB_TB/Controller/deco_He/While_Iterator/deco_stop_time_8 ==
  note: Model: RB_TB/Controller/deco_He/While_Iterator/deco_stop_time_X
  In1 : Inport  Port=1  LatchInput=off
  In2 : Inport  Port=2  LatchInput=off
  >10e-300 : Saturate  UpperLimit=inf  LowerLimit=10e-320
  >10e-320 : Switch  Threshold=10e-320
  BS1 : BusSelector  DialogController=Simulink.DDGSource_Bus  OutputSignals=He_k,Pt_stop,He_b,M0
  BS2 : BusSelector  DialogController=Simulink.DDGSource_Bus  OutputSignals=Pstop_next,Palv_next,stop_time
  Constant : Constant
  Mem : Memory  InheritSampleTime=on
  Mux1 : Mux  Inputs=2
  Mux2 : Mux
  Mux3 : Mux  Inputs=2
  Mux4 : Mux  Inputs=3
  Mux5 : Mux  Inputs=3
  fcn(14)1 : Fcn  Expr=log(u(1))
  fcn(14)2 : Fcn  Expr=u(1)-u(2)
  fcn(14)4 : Fcn  Expr=(u(2)-u(3))/u(1)
  fcn(14)5 : Fcn  Expr=-u(2)/u(1)
  fcn1 : Fcn  Expr=u(2)+u(3)/u(1)
  fcn2 : Fcn  Expr=u(3)+(u(2)-u(3))*exp(-u(1)*u(4))
  Pt_new : Outport
  deco_stop_time : Outport  Port=2
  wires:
  >10e-300/1 -> Mux5/1
  Mux5/1 -> fcn(14)4/1
  fcn(14)2/1 -> >10e-300/1
  Mux3/1 -> fcn(14)2/1
  BS2/1 -> Mux4/3  "<Pstop_next>"
  Constant/1 -> >10e-320/3
  fcn(14)4/1 -> >10e-320/1, >10e-320/2
  fcn(14)1/1 -> Mux1/2
  >10e-320/1 -> fcn(14)1/1
  Mux4/1 -> fcn1/1
  fcn(14)5/1 -> deco_stop_time/1  "deco_stop_time"
  fcn1/1 -> Mux5/2  "M_next"
  BS2/2 -> Mux3/2, Mux5/3, Mux2/3  "<Palv_next>"
  BS1/1 -> Mux1/1, Mux2/1  "<He_k>"
  Mux1/1 -> fcn(14)5/1
  BS1/4 -> Mux4/2  "<M0>"
  BS1/3 -> Mux4/1  "<He_b>"
  In1/1 -> BS1/1
  BS1/2 -> Mux3/1, Mux2/2  "<Pt_stop>"
  Mux2/1 -> fcn2/1
  fcn2/1 -> Mem/1
  BS2/3 -> Mux2/4  "<stop_time>"
  Mem/1 -> Pt_new/1
  In2/1 -> BS2/1

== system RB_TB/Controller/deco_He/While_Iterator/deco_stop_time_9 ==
  note: Model: RB_TB/Controller/deco_He/While_Iterator/deco_stop_time_X
  In1 : Inport  Port=1  LatchInput=off
  In2 : Inport  Port=2  LatchInput=off
  >10e-300 : Saturate  UpperLimit=inf  LowerLimit=10e-320
  >10e-320 : Switch  Threshold=10e-320
  BS1 : BusSelector  DialogController=Simulink.DDGSource_Bus  OutputSignals=He_k,Pt_stop,He_b,M0
  BS2 : BusSelector  DialogController=Simulink.DDGSource_Bus  OutputSignals=Pstop_next,Palv_next,stop_time
  Constant : Constant
  Mem : Memory  InheritSampleTime=on
  Mux1 : Mux  Inputs=2
  Mux2 : Mux
  Mux3 : Mux  Inputs=2
  Mux4 : Mux  Inputs=3
  Mux5 : Mux  Inputs=3
  fcn(14)1 : Fcn  Expr=log(u(1))
  fcn(14)2 : Fcn  Expr=u(1)-u(2)
  fcn(14)4 : Fcn  Expr=(u(2)-u(3))/u(1)
  fcn(14)5 : Fcn  Expr=-u(2)/u(1)
  fcn1 : Fcn  Expr=u(2)+u(3)/u(1)
  fcn2 : Fcn  Expr=u(3)+(u(2)-u(3))*exp(-u(1)*u(4))
  Pt_new : Outport
  deco_stop_time : Outport  Port=2
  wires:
  In2/1 -> BS2/1
  Mem/1 -> Pt_new/1
  BS2/3 -> Mux2/4  "<stop_time>"
  fcn2/1 -> Mem/1
  Mux2/1 -> fcn2/1
  BS1/2 -> Mux2/2, Mux3/1  "<Pt_stop>"
  In1/1 -> BS1/1
  BS1/3 -> Mux4/1  "<He_b>"
  BS1/4 -> Mux4/2  "<M0>"
  Mux1/1 -> fcn(14)5/1
  BS1/1 -> Mux2/1, Mux1/1  "<He_k>"
  BS2/2 -> Mux2/3, Mux5/3, Mux3/2  "<Palv_next>"
  fcn1/1 -> Mux5/2  "M_next"
  fcn(14)5/1 -> deco_stop_time/1  "deco_stop_time"
  Mux4/1 -> fcn1/1
  >10e-320/1 -> fcn(14)1/1
  fcn(14)1/1 -> Mux1/2
  fcn(14)4/1 -> >10e-320/2, >10e-320/1
  Constant/1 -> >10e-320/3
  BS2/1 -> Mux4/3  "<Pstop_next>"
  Mux3/1 -> fcn(14)2/1
  fcn(14)2/1 -> >10e-300/1
  Mux5/1 -> fcn(14)4/1
  >10e-300/1 -> Mux5/1

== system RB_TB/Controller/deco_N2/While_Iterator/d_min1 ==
  note: Model: RB_TB/Controller/deco_N2/While_Iterator/d_minX
  Pt_new : Inport  Port=1  LatchInput=off
  In1 : Inport  Port=2  LatchInput=off
  In2 : Inport  Port=3  LatchInput=off
  BC : BusCreator  DialogController=Simulink.DDGSource_Bus
  BS1 : BusSelector  DialogController=Simulink.DDGSource_Bus  OutputSignals=N2_b,M0,N2_k,Pt
  BS2 : BusSelector  DialogController=Simulink.DDGSource_Bus  OutputSignals=rate_asc,asc_time,while,cnc_N2,Palv_next,Palv
  Mux2 : Mux  Inputs=6
  Product2 : Product
  Sum1 : Sum  Inputs=-+|
  Switch : Switch  Threshold=2
  Switch1 : Switch  Threshold=2
  fnc : Fcn  Expr=u(6)-u(5)*u(2)*(u(3)-1/u(1))-(u(6)-u(4)+u(5)*u(2)/u(1))*exp(-u(1)*u(3))
  prod : Gain  Gain=10
  bus1 : Outport
  d_min : Outport  Port=2
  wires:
  BS1/3 -> Mux2/1, BC/3  "<N2_k>"
  BS1/1 -> prod/1, BC/1  "<N2_b>"
  BS1/2 -> Sum1/1, BC/2  "<M0>"
  Mux2/1 -> fnc/1
  fnc/1 -> BC/4  "Pt_stop"
  BS2/2 -> Mux2/3  "<asc_time>"
  BS2/4 -> Mux2/5  "<cnc_N2>"
  In1/1 -> BS1/1
  Sum1/1 -> Product2/2
  prod/1 -> Product2/1
  Product2/1 -> d_min/1
  BC/1 -> bus1/1
  Switch/1 -> Sum1/2, Mux2/4  "Pt"
  BS1/4 -> Switch/3  "<Pt>"
  Pt_new/1 -> Switch/1
  Switch1/1 -> Mux2/6
  BS2/6 -> Switch1/3  "<Palv>"
  BS2/3 -> Switch/2, Switch1/2  "<while>"
  BS2/5 -> Switch1/1  "<Palv_next>"
  In2/1 -> BS2/1
  BS2/1 -> Mux2/2  "<rate_asc>"

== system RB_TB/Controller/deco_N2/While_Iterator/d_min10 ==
  note: Model: RB_TB/Controller/deco_N2/While_Iterator/d_minX
  Pt_new : Inport  Port=1  LatchInput=off
  In1 : Inport  Port=2  LatchInput=off
  In2 : Inport  Port=3  LatchInput=off
  BC : BusCreator  DialogController=Simulink.DDGSource_Bus
  BS1 : BusSelector  DialogController=Simulink.DDGSource_Bus  OutputSignals=N2_b,M0,N2_k,Pt
  BS2 : BusSelector  DialogController=Simulink.DDGSource_Bus  OutputSignals=rate_asc,asc_time,while,cnc_N2,Palv_next,Palv
  Mux2 : Mux  Inputs=6
  Product2 : Product
  Sum1 : Sum  Inputs=-+|
  Switch : Switch  Threshold=2
  Switch1 : Switch  Threshold=2
  fnc : Fcn  Expr=u(6)-u(5)*u(2)*(u(3)-1/u(1))-(u(6)-u(4)+u(5)*u(2)/u(1))*exp(-u(1)*u(3))
  prod : Gain  Gain=10
  bus1 : Outport
  d_min : Outport  Port=2
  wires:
  BS2/1 -> Mux2/2  "<rate_asc>"
  In2/1 -> BS2/1
  BS2/5 -> Switch1/1  "<Palv_next>"
  BS2/3 -> Switch1/2, Switch/2  "<while>"
  BS2/6 -> Switch1/3  "<Palv>"
  Switch1/1 -> Mux2/6
  Pt_new/1 -> Switch/1
  BS1/4 -> Switch/3  "<Pt>"
  Switch/1 -> Mux2/4, Sum1/2  "Pt"
  BC/1 -> bus1/1
  Product2/1 -> d_min/1
  prod/1 -> Product2/1
  Sum1/1 -> Product2/2
  In1/1 -> BS1/1
  BS2/4 -> Mux2/5  "<cnc_N2>"
  BS2/2 -> Mux2/3  "<asc_time>"
  fnc/1 -> BC/4  "Pt_stop"
  Mux2/1 -> fnc/1
  BS1/2 -> BC/2, Sum1/1  "<M0>"
  BS1/1 -> BC/1, prod/1  "<N2_b>"
  BS1/3 -> BC/3, Mux2/1  "<N2_k>"

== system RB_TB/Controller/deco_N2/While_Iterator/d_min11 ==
  note: Model: RB_TB/Controller/deco_N2/While_Iterator/d_minX
  Pt_new : Inport  Port=1  LatchInput=off
  In1 : Inport  Port=2  LatchInput=off
  In2 : Inport  Port=3  LatchInput=off
  BC : BusCreator  DialogController=Simulink.DDGSource_Bus
  BS1 : BusSelector  DialogController=Simulink.DDGSource_Bus  OutputSignals=N2_b,M0,N2_k,Pt
  BS2 : BusSelector  DialogController=Simulink.DDGSource_Bus  OutputSignals=rate_asc,asc_time,while,cnc_N2,Palv_next,Palv
  Mux2 : Mux  Inputs=6
  Product2 : Product
  Sum1 : Sum  Inputs=-+|
  Switch : Switch  Threshold=2
  Switch1 : Switch  Threshold=2
  fnc : Fcn  Expr=u(6)-u(5)*u(2)*(u(3)-1/u(1))-(u(6)-u(4)+u(5)*u(2)/u(1))*exp(-u(1)*u(3))
  prod : Gain  Gain=10
  bus1 : Outport
  d_min : Outport  Port=2
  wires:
  BS1/3 -> Mux2/1, BC/3  "<N2_k>"
  BS1/1 -> prod/1, BC/1  "<N2_b>"
  BS1/2 -> Sum1/1, BC/2  "<M0>"
  Mux2/1 -> fnc/1
  fnc/1 -> BC/4  "Pt_stop"
  BS2/2 -> Mux2/3  "<asc_time>"
  BS2/4 -> Mux2/5  "<cnc_N2>"
  In1/1 -> BS1/1
  Sum1/1 -> Product2/2
  prod/1 -> Product2/1
  Product2/1 -> d_min/1
  BC/1 -> bus1/1
  Switch/1 -> Sum1/2, Mux2/4  "Pt"
  BS1/4 -> Switch/3  "<Pt>"
  Pt_new/1 -> Switch/1
  Switch1/1 -> Mux2/6
  BS2/6 -> Switch1/3  "<Palv>"
  BS2/3 -> Switch/2, Switch1/2  "<while>"
  BS2/5 -> Switch1/1  "<Palv_next>"
  In2/1 -> BS2/1
  BS2/1 -> Mux2/2  "<rate_asc>"

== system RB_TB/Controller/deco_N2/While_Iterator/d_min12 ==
  note: Model: RB_TB/Controller/deco_N2/While_Iterator/d_minX
  Pt_new : Inport  Port=1  LatchInput=off
  In1 : Inport  Port=2  LatchInput=off
  In2 : Inport  Port=3  LatchInput=off
  BC : BusCreator  DialogController=Simulink.DDGSource_Bus
  BS1 : BusSelector  DialogController=Simulink.DDGSource_Bus  OutputSignals=N2_b,M0,N2_k,Pt
  BS2 : BusSelector  DialogController=Simulink.DDGSource_Bus  OutputSignals=rate_asc,asc_time,while,cnc_N2,Palv_next,Palv
  Mux2 : Mux  Inputs=6
  Product2 : Product
  Sum1 : Sum  Inputs=-+|
  Switch : Switch  Threshold=2
  Switch1 : Switch  Threshold=2
  fnc : Fcn  Expr=u(6)-u(5)*u(2)*(u(3)-1/u(1))-(u(6)-u(4)+u(5)*u(2)/u(1))*exp(-u(1)*u(3))
  prod : Gain  Gain=10
  bus1 : Outport
  d_min : Outport  Port=2
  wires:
  BS2/1 -> Mux2/2  "<rate_asc>"
  In2/1 -> BS2/1
  BS2/5 -> Switch1/1  "<Palv_next>"
  BS2/3 -> Switch1/2, Switch/2  "<while>"
  BS2/6 -> Switch1/3  "<Palv>"
  Switch1/1 -> Mux2/6
  Pt_new/1 -> Switch/1
  BS1/4 -> Switch/3  "<Pt>"
  Switch/1 -> Mux2/4, Sum1/2  "Pt"
  BC/1 -> bus1/1
  Product2/1 -> d_min/1
  prod/1 -> Product2/1
  Sum1/1 -> Product2/2
  In1/1 -> BS1/1
  BS2/4 -> Mux2/5  "<cnc_N2>"
  BS2/2 -> Mux2/3  "<asc_time>"
  fnc/1 -> BC/4  "Pt_stop"
  Mux2/1 -> fnc/1
  BS1/2 -> BC/2, Sum1/1  "<M0>"
  BS1/1 -> BC/1, prod/1  "<N2_b>"
  BS1/3 -> BC/3, Mux2/1  "<N2_k>"

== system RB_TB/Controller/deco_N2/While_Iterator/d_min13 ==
  note: Model: RB_TB/Controller/deco_N2/While_Iterator/d_minX
  Pt_new : Inport  Port=1  LatchInput=off
  In1 : Inport  Port=2  LatchInput=off
  In2 : Inport  Port=3  LatchInput=off
  BC : BusCreator  DialogController=Simulink.DDGSource_Bus
  BS1 : BusSelector  DialogController=Simulink.DDGSource_Bus  OutputSignals=N2_b,M0,N2_k,Pt
  BS2 : BusSelector  DialogController=Simulink.DDGSource_Bus  OutputSignals=rate_asc,asc_time,while,cnc_N2,Palv_next,Palv
  Mux2 : Mux  Inputs=6
  Product2 : Product
  Sum1 : Sum  Inputs=-+|
  Switch : Switch  Threshold=2
  Switch1 : Switch  Threshold=2
  fnc : Fcn  Expr=u(6)-u(5)*u(2)*(u(3)-1/u(1))-(u(6)-u(4)+u(5)*u(2)/u(1))*exp(-u(1)*u(3))
  prod : Gain  Gain=10
  bus1 : Outport
  d_min : Outport  Port=2
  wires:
  BS1/3 -> Mux2/1, BC/3  "<N2_k>"
  BS1/1 -> prod/1, BC/1  "<N2_b>"
  BS1/2 -> Sum1/1, BC/2  "<M0>"
  Mux2/1 -> fnc/1
  fnc/1 -> BC/4  "Pt_stop"
  BS2/2 -> Mux2/3  "<asc_time>"
  BS2/4 -> Mux2/5  "<cnc_N2>"
  In1/1 -> BS1/1
  Sum1/1 -> Product2/2
  prod/1 -> Product2/1
  Product2/1 -> d_min/1
  BC/1 -> bus1/1
  Switch/1 -> Sum1/2, Mux2/4  "Pt"
  BS1/4 -> Switch/3  "<Pt>"
  Pt_new/1 -> Switch/1
  Switch1/1 -> Mux2/6
  BS2/6 -> Switch1/3  "<Palv>"
  BS2/3 -> Switch/2, Switch1/2  "<while>"
  BS2/5 -> Switch1/1  "<Palv_next>"
  In2/1 -> BS2/1
  BS2/1 -> Mux2/2  "<rate_asc>"

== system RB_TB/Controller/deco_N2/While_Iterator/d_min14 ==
  note: Model: RB_TB/Controller/deco_N2/While_Iterator/d_minX
  Pt_new : Inport  Port=1  LatchInput=off
  In1 : Inport  Port=2  LatchInput=off
  In2 : Inport  Port=3  LatchInput=off
  BC : BusCreator  DialogController=Simulink.DDGSource_Bus
  BS1 : BusSelector  DialogController=Simulink.DDGSource_Bus  OutputSignals=N2_b,M0,N2_k,Pt
  BS2 : BusSelector  DialogController=Simulink.DDGSource_Bus  OutputSignals=rate_asc,asc_time,while,cnc_N2,Palv_next,Palv
  Mux2 : Mux  Inputs=6
  Product2 : Product
  Sum1 : Sum  Inputs=-+|
  Switch : Switch  Threshold=2
  Switch1 : Switch  Threshold=2
  fnc : Fcn  Expr=u(6)-u(5)*u(2)*(u(3)-1/u(1))-(u(6)-u(4)+u(5)*u(2)/u(1))*exp(-u(1)*u(3))
  prod : Gain  Gain=10
  bus1 : Outport
  d_min : Outport  Port=2
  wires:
  BS2/1 -> Mux2/2  "<rate_asc>"
  In2/1 -> BS2/1
  BS2/5 -> Switch1/1  "<Palv_next>"
  BS2/3 -> Switch1/2, Switch/2  "<while>"
  BS2/6 -> Switch1/3  "<Palv>"
  Switch1/1 -> Mux2/6
  Pt_new/1 -> Switch/1
  BS1/4 -> Switch/3  "<Pt>"
  Switch/1 -> Mux2/4, Sum1/2  "Pt"
  BC/1 -> bus1/1
  Product2/1 -> d_min/1
  prod/1 -> Product2/1
  Sum1/1 -> Product2/2
  In1/1 -> BS1/1
  BS2/4 -> Mux2/5  "<cnc_N2>"
  BS2/2 -> Mux2/3  "<asc_time>"
  fnc/1 -> BC/4  "Pt_stop"
  Mux2/1 -> fnc/1
  BS1/2 -> BC/2, Sum1/1  "<M0>"
  BS1/1 -> BC/1, prod/1  "<N2_b>"
  BS1/3 -> BC/3, Mux2/1  "<N2_k>"

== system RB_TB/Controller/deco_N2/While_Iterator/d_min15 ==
  note: Model: RB_TB/Controller/deco_N2/While_Iterator/d_minX
  Pt_new : Inport  Port=1  LatchInput=off
  In1 : Inport  Port=2  LatchInput=off
  In2 : Inport  Port=3  LatchInput=off
  BC : BusCreator  DialogController=Simulink.DDGSource_Bus
  BS1 : BusSelector  DialogController=Simulink.DDGSource_Bus  OutputSignals=N2_b,M0,N2_k,Pt
  BS2 : BusSelector  DialogController=Simulink.DDGSource_Bus  OutputSignals=rate_asc,asc_time,while,cnc_N2,Palv_next,Palv
  Mux2 : Mux  Inputs=6
  Product2 : Product
  Sum1 : Sum  Inputs=-+|
  Switch : Switch  Threshold=2
  Switch1 : Switch  Threshold=2
  fnc : Fcn  Expr=u(6)-u(5)*u(2)*(u(3)-1/u(1))-(u(6)-u(4)+u(5)*u(2)/u(1))*exp(-u(1)*u(3))
  prod : Gain  Gain=10
  bus1 : Outport
  d_min : Outport  Port=2
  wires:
  BS1/3 -> Mux2/1, BC/3  "<N2_k>"
  BS1/1 -> prod/1, BC/1  "<N2_b>"
  BS1/2 -> Sum1/1, BC/2  "<M0>"
  Mux2/1 -> fnc/1
  fnc/1 -> BC/4  "Pt_stop"
  BS2/2 -> Mux2/3  "<asc_time>"
  BS2/4 -> Mux2/5  "<cnc_N2>"
  In1/1 -> BS1/1
  Sum1/1 -> Product2/2
  prod/1 -> Product2/1
  Product2/1 -> d_min/1
  BC/1 -> bus1/1
  Switch/1 -> Sum1/2, Mux2/4  "Pt"
  BS1/4 -> Switch/3  "<Pt>"
  Pt_new/1 -> Switch/1
  Switch1/1 -> Mux2/6
  BS2/6 -> Switch1/3  "<Palv>"
  BS2/3 -> Switch/2, Switch1/2  "<while>"
  BS2/5 -> Switch1/1  "<Palv_next>"
  In2/1 -> BS2/1
  BS2/1 -> Mux2/2  "<rate_asc>"

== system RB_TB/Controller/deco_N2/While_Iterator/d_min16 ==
  note: Model: RB_TB/Controller/deco_N2/While_Iterator/d_minX
  Pt_new : Inport  Port=1  LatchInput=off
  In1 : Inport  Port=2  LatchInput=off
  In2 : Inport  Port=3  LatchInput=off
  BC : BusCreator  DialogController=Simulink.DDGSource_Bus
  BS1 : BusSelector  DialogController=Simulink.DDGSource_Bus  OutputSignals=N2_b,M0,N2_k,Pt
  BS2 : BusSelector  DialogController=Simulink.DDGSource_Bus  OutputSignals=rate_asc,asc_time,while,cnc_N2,Palv_next,Palv
  Mux2 : Mux  Inputs=6
  Product2 : Product
  Sum1 : Sum  Inputs=-+|
  Switch : Switch  Threshold=2
  Switch1 : Switch  Threshold=2
  fnc : Fcn  Expr=u(6)-u(5)*u(2)*(u(3)-1/u(1))-(u(6)-u(4)+u(5)*u(2)/u(1))*exp(-u(1)*u(3))
  prod : Gain  Gain=10
  bus1 : Outport
  d_min : Outport  Port=2
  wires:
  BS2/1 -> Mux2/2  "<rate_asc>"
  In2/1 -> BS2/1
  BS2/5 -> Switch1/1  "<Palv_next>"
  BS2/3 -> Switch1/2, Switch/2  "<while>"
  BS2/6 -> Switch1/3  "<Palv>"
  Switch1/1 -> Mux2/6
  Pt_new/1 -> Switch/1
  BS1/4 -> Switch/3  "<Pt>"
  Switch/1 -> Mux2/4, Sum1/2  "Pt"
  BC/1 -> bus1/1
  Product2/1 -> d_min/1
  prod/1 -> Product2/1
  Sum1/1 -> Product2/2
  In1/1 -> BS1/1
  BS2/4 -> Mux2/5  "<cnc_N2>"
  BS2/2 -> Mux2/3  "<asc_time>"
  fnc/1 -> BC/4  "Pt_stop"
  Mux2/1 -> fnc/1
  BS1/2 -> BC/2, Sum1/1  "<M0>"
  BS1/1 -> BC/1, prod/1  "<N2_b>"
  BS1/3 -> BC/3, Mux2/1  "<N2_k>"

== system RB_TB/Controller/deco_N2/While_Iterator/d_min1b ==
  note: Model: RB_TB/Controller/deco_N2/While_Iterator/d_minX
  Pt_new : Inport  Port=1  LatchInput=off
  In1 : Inport  Port=2  LatchInput=off
  In2 : Inport  Port=3  LatchInput=off
  BC : BusCreator  DialogController=Simulink.DDGSource_Bus
  BS1 : BusSelector  DialogController=Simulink.DDGSource_Bus  OutputSignals=N2_b,M0,N2_k,Pt
  BS2 : BusSelector  DialogController=Simulink.DDGSource_Bus  OutputSignals=rate_asc,asc_time,while,cnc_N2,Palv_next,Palv
  Mux2 : Mux  Inputs=6
  Product2 : Product
  Sum1 : Sum  Inputs=-+|
  Switch : Switch  Threshold=2
  Switch1 : Switch  Threshold=2
  fnc : Fcn  Expr=u(6)-u(5)*u(2)*(u(3)-1/u(1))-(u(6)-u(4)+u(5)*u(2)/u(1))*exp(-u(1)*u(3))
  prod : Gain  Gain=10
  bus1 : Outport
  d_min : Outport  Port=2
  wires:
  BS1/3 -> Mux2/1, BC/3  "<N2_k>"
  BS1/1 -> prod/1, BC/1  "<N2_b>"
  BS1/2 -> Sum1/1, BC/2  "<M0>"
  Mux2/1 -> fnc/1
  fnc/1 -> BC/4  "Pt_stop"
  BS2/2 -> Mux2/3  "<asc_time>"
  BS2/4 -> Mux2/5  "<cnc_N2>"
  In1/1 -> BS1/1
  Sum1/1 -> Product2/2
  prod/1 -> Product2/1
  Product2/1 -> d_min/1
  BC/1 -> bus1/1
  Switch/1 -> Sum1/2, Mux2/4  "Pt"
  BS1/4 -> Switch/3  "<Pt>"
  Pt_new/1 -> Switch/1
  Switch1/1 -> Mux2/6
  BS2/6 -> Switch1/3  "<Palv>"
  BS2/3 -> Switch/2, Switch1/2  "<while>"
  BS2/5 -> Switch1/1  "<Palv_next>"
  In2/1 -> BS2/1
  BS2/1 -> Mux2/2  "<rate_asc>"

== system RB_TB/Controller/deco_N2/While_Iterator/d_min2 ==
  note: Model: RB_TB/Controller/deco_N2/While_Iterator/d_minX
  Pt_new : Inport  Port=1  LatchInput=off
  In1 : Inport  Port=2  LatchInput=off
  In2 : Inport  Port=3  LatchInput=off
  BC : BusCreator  DialogController=Simulink.DDGSource_Bus
  BS1 : BusSelector  DialogController=Simulink.DDGSource_Bus  OutputSignals=N2_b,M0,N2_k,Pt
  BS2 : BusSelector  DialogController=Simulink.DDGSource_Bus  OutputSignals=rate_asc,asc_time,while,cnc_N2,Palv_next,Palv
  Mux2 : Mux  Inputs=6
  Product2 : Product
  Sum1 : Sum  Inputs=-+|
  Switch : Switch  Threshold=2
  Switch1 : Switch  Threshold=2
  fnc : Fcn  Expr=u(6)-u(5)*u(2)*(u(3)-1/u(1))-(u(6)-u(4)+u(5)*u(2)/u(1))*exp(-u(1)*u(3))
  prod : Gain  Gain=10
  bus1 : Outport
  d_min : Outport  Port=2
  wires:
  BS2/1 -> Mux2/2  "<rate_asc>"
  In2/1 -> BS2/1
  BS2/5 -> Switch1/1  "<Palv_next>"
  BS2/3 -> Switch1/2, Switch/2  "<while>"
  BS2/6 -> Switch1/3  "<Palv>"
  Switch1/1 -> Mux2/6
  Pt_new/1 -> Switch/1
  BS1/4 -> Switch/3  "<Pt>"
  Switch/1 -> Mux2/4, Sum1/2  "Pt"
  BC/1 -> bus1/1
  Product2/1 -> d_min/1
  prod/1 -> Product2/1
  Sum1/1 -> Product2/2
  In1/1 -> BS1/1
  BS2/4 -> Mux2/5  "<cnc_N2>"
  BS2/2 -> Mux2/3  "<asc_time>"
  fnc/1 -> BC/4  "Pt_stop"
  Mux2/1 -> fnc/1
  BS1/2 -> BC/2, Sum1/1  "<M0>"
  BS1/1 -> BC/1, prod/1  "<N2_b>"
  BS1/3 -> BC/3, Mux2/1  "<N2_k>"

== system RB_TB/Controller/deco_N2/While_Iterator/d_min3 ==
  note: Model: RB_TB/Controller/deco_N2/While_Iterator/d_minX
  Pt_new : Inport  Port=1  LatchInput=off
  In1 : Inport  Port=2  LatchInput=off
  In2 : Inport  Port=3  LatchInput=off
  BC : BusCreator  DialogController=Simulink.DDGSource_Bus
  BS1 : BusSelector  DialogController=Simulink.DDGSource_Bus  OutputSignals=N2_b,M0,N2_k,Pt
  BS2 : BusSelector  DialogController=Simulink.DDGSource_Bus  OutputSignals=rate_asc,asc_time,while,cnc_N2,Palv_next,Palv
  Mux2 : Mux  Inputs=6
  Product2 : Product
  Sum1 : Sum  Inputs=-+|
  Switch : Switch  Threshold=2
  Switch1 : Switch  Threshold=2
  fnc : Fcn  Expr=u(6)-u(5)*u(2)*(u(3)-1/u(1))-(u(6)-u(4)+u(5)*u(2)/u(1))*exp(-u(1)*u(3))
  prod : Gain  Gain=10
  bus1 : Outport
  d_min : Outport  Port=2
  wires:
  BS1/3 -> Mux2/1, BC/3  "<N2_k>"
  BS1/1 -> prod/1, BC/1  "<N2_b>"
  BS1/2 -> Sum1/1, BC/2  "<M0>"
  Mux2/1 -> fnc/1
  fnc/1 -> BC/4  "Pt_stop"
  BS2/2 -> Mux2/3  "<asc_time>"
  BS2/4 -> Mux2/5  "<cnc_N2>"
  In1/1 -> BS1/1
  Sum1/1 -> Product2/2
  prod/1 -> Product2/1
  Product2/1 -> d_min/1
  BC/1 -> bus1/1
  Switch/1 -> Sum1/2, Mux2/4  "Pt"
  BS1/4 -> Switch/3  "<Pt>"
  Pt_new/1 -> Switch/1
  Switch1/1 -> Mux2/6
  BS2/6 -> Switch1/3  "<Palv>"
  BS2/3 -> Switch/2, Switch1/2  "<while>"
  BS2/5 -> Switch1/1  "<Palv_next>"
  In2/1 -> BS2/1
  BS2/1 -> Mux2/2  "<rate_asc>"

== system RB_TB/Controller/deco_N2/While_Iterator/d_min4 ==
  note: Model: RB_TB/Controller/deco_N2/While_Iterator/d_minX
  Pt_new : Inport  Port=1  LatchInput=off
  In1 : Inport  Port=2  LatchInput=off
  In2 : Inport  Port=3  LatchInput=off
  BC : BusCreator  DialogController=Simulink.DDGSource_Bus
  BS1 : BusSelector  DialogController=Simulink.DDGSource_Bus  OutputSignals=N2_b,M0,N2_k,Pt
  BS2 : BusSelector  DialogController=Simulink.DDGSource_Bus  OutputSignals=rate_asc,asc_time,while,cnc_N2,Palv_next,Palv
  Mux2 : Mux  Inputs=6
  Product2 : Product
  Sum1 : Sum  Inputs=-+|
  Switch : Switch  Threshold=2
  Switch1 : Switch  Threshold=2
  fnc : Fcn  Expr=u(6)-u(5)*u(2)*(u(3)-1/u(1))-(u(6)-u(4)+u(5)*u(2)/u(1))*exp(-u(1)*u(3))
  prod : Gain  Gain=10
  bus1 : Outport
  d_min : Outport  Port=2
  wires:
  BS2/1 -> Mux2/2  "<rate_asc>"
  In2/1 -> BS2/1
  BS2/5 -> Switch1/1  "<Palv_next>"
  BS2/3 -> Switch1/2, Switch/2  "<while>"
  BS2/6 -> Switch1/3  "<Palv>"
  Switch1/1 -> Mux2/6
  Pt_new/1 -> Switch/1
  BS1/4 -> Switch/3  "<Pt>"
  Switch/1 -> Mux2/4, Sum1/2  "Pt"
  BC/1 -> bus1/1
  Product2/1 -> d_min/1
  prod/1 -> Product2/1
  Sum1/1 -> Product2/2
  In1/1 -> BS1/1
  BS2/4 -> Mux2/5  "<cnc_N2>"
  BS2/2 -> Mux2/3  "<asc_time>"
  fnc/1 -> BC/4  "Pt_stop"
  Mux2/1 -> fnc/1
  BS1/2 -> BC/2, Sum1/1  "<M0>"
  BS1/1 -> BC/1, prod/1  "<N2_b>"
  BS1/3 -> BC/3, Mux2/1  "<N2_k>"

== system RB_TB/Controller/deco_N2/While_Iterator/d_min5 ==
  note: Model: RB_TB/Controller/deco_N2/While_Iterator/d_minX
  Pt_new : Inport  Port=1  LatchInput=off
  In1 : Inport  Port=2  LatchInput=off
  In2 : Inport  Port=3  LatchInput=off
  BC : BusCreator  DialogController=Simulink.DDGSource_Bus
  BS1 : BusSelector  DialogController=Simulink.DDGSource_Bus  OutputSignals=N2_b,M0,N2_k,Pt
  BS2 : BusSelector  DialogController=Simulink.DDGSource_Bus  OutputSignals=rate_asc,asc_time,while,cnc_N2,Palv_next,Palv
  Mux2 : Mux  Inputs=6
  Product2 : Product
  Sum1 : Sum  Inputs=-+|
  Switch : Switch  Threshold=2
  Switch1 : Switch  Threshold=2
  fnc : Fcn  Expr=u(6)-u(5)*u(2)*(u(3)-1/u(1))-(u(6)-u(4)+u(5)*u(2)/u(1))*exp(-u(1)*u(3))
  prod : Gain  Gain=10
  bus1 : Outport
  d_min : Outport  Port=2
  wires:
  BS1/3 -> Mux2/1, BC/3  "<N2_k>"
  BS1/1 -> prod/1, BC/1  "<N2_b>"
  BS1/2 -> Sum1/1, BC/2  "<M0>"
  Mux2/1 -> fnc/1
  fnc/1 -> BC/4  "Pt_stop"
  BS2/2 -> Mux2/3  "<asc_time>"
  BS2/4 -> Mux2/5  "<cnc_N2>"
  In1/1 -> BS1/1
  Sum1/1 -> Product2/2
  prod/1 -> Product2/1
  Product2/1 -> d_min/1
  BC/1 -> bus1/1
  Switch/1 -> Sum1/2, Mux2/4  "Pt"
  BS1/4 -> Switch/3  "<Pt>"
  Pt_new/1 -> Switch/1
  Switch1/1 -> Mux2/6
  BS2/6 -> Switch1/3  "<Palv>"
  BS2/3 -> Switch/2, Switch1/2  "<while>"
  BS2/5 -> Switch1/1  "<Palv_next>"
  In2/1 -> BS2/1
  BS2/1 -> Mux2/2  "<rate_asc>"
